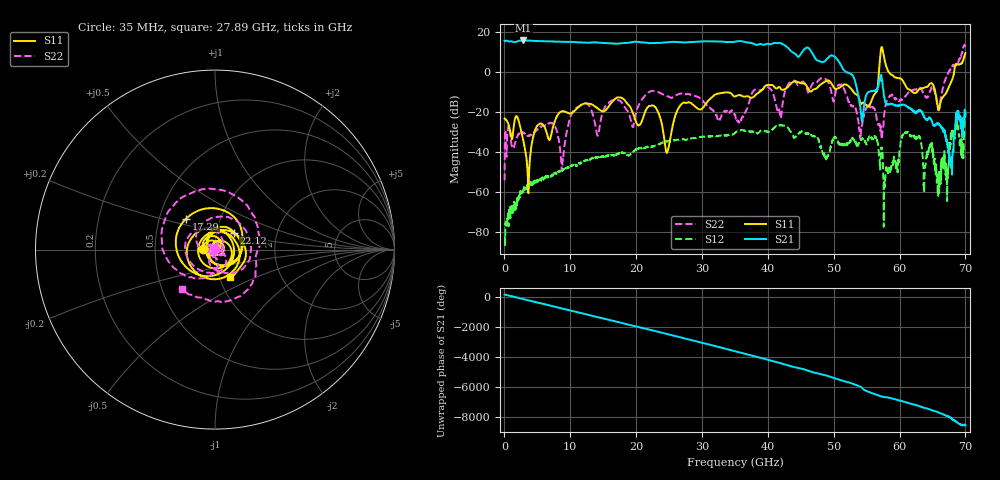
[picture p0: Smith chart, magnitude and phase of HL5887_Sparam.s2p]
! 11/28/2022 3:28:05 PM
! H:\PRODUCTION_DATA\TEMP_S2P.S2P
! CHANNEL.1
! TR.MEASUREMENT
! CORRECTED.DATA
# GHZ S RI R 50.0
! FREQ.GHZ  S11RE  S11IM  S21RE  S21IM  S12RE  S12IM  S22RE  S22IM
!; PortSelection: Port_12
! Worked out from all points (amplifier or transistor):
!   2000 points, 35 MHz to 70 GHz, reference 50 ohm
!   highest |S21| = 15.9 dB at 2.87 GHz (marker M1)
!   |S21| within 3 dB of that: start of sweep to 42.81 GHz
!   unconditionally stable (mu >= 1): start of sweep to 56.86 GHz; 58.4 GHz to 67.43 GHz
!   at 11.69 GHz: K = 15.86, MAG = 15.1 dB, |S12| = -45.3 dB
!   at 35.03 GHz: K = 2.67, MAG = 15.7 dB, |S12| = -30.2 dB
!   at 70 GHz: K = 7430.81, MSG = -0.6 dB, |S12| = -19.4 dB
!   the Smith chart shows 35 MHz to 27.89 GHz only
!   S11 on the Smith chart (normalised r, x): 35 MHz: 0.87, +0.01; 17.29 GHz: 0.69, +0.25; 22.12 GHz: 1.21, +0.24; 27.89 GHz: 1.13, -0.36
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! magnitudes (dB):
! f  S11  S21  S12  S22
! 35 MHz  -23.2  15.9  -82.0  -54.1
! 2.87 GHz  -34.1  15.9  -58.2  -30.2
! 3.64 GHz  -60.5  15.9  -57.3  -31.8
! 4.97 GHz  -26.9  15.7  -53.8  -28.7
! 7.28 GHz  -28.7  15.4  -51.0  -25.5
! 8.785 GHz  -19.5  15.3  -49.5  -47.5
! 11.72 GHz  -16.1  14.9  -44.9  -16.4
! 14.18 GHz  -18.1  14.9  -42.6  -31.7
! 17.29 GHz  -12.5  14.3  -40.6  -14.0
! 19.46 GHz  -19.9  15.2  -40.2  -27.4
! 22.12 GHz  -16.9  14.6  -37.6  -9.6
! 23.38 GHz  -20.2  14.7  -36.2  -9.9
! 24.75 GHz  -40.0  15.0  -34.5  -11.9
! 27.89 GHz  -15.0  15.1  -33.3  -10.9
! 35.03 GHz  -12.1  15.4  -30.2  -21.1
! 46.69 GHz  -9.4  9.9  -31.6  -6.3
! 54.04 GHz  -15.3  -17.6  -34.0  -31.5
! 58.34 GHz  0.2  -15.9  -48.3  -12.5
! 61.11 GHz  -7.8  -17.1  -30.3  -11.2
! 65.97 GHz  -18.8  -26.2  -60.5  -18.8
! 67.76 GHz  -5.3  -46.0  -33.6  2.1
! 70 GHz  9.6  -20.6  -19.4  12.8
